FUNCTION_BLOCK FB84
TITLE =Move With Velocity
//*****************************************************************************
//* maxon motor ag
//* R&D
//* all rights reserved
//*****************************************************************************
//* Summary:  Move with target velocity
//*
//* Remarks:
//*
//* Created under: STEP7 REV5.2+SP1
//*****************************************************************************
//* History:
//* 19.05.2004 | INA   first release
//*
//*
//*****************************************************************************
//

AUTHOR:INA
FAMILY:ProVeloM
NAME:MoveWVel
VERSION:00.01


VAR_INPUT

Write : BOOL //A rising edge start the command

  NodeID : BYTE //Adress of the maxon device

  TargetVelocity : DINT //Target Velocity

END_VAR
VAR_OUTPUT
  Done : BOOL //Data valid flag is TRUE if data were available

  Err : BOOL //Error flag is TRUE if an Error has occured, see ErrNo for more details

  ErrNo : DINT //Contains detailed error information

END_VAR
VAR
  xEdgeMerker : BOOL //Edge Merker

  xEdgeFlag : BOOL //Edge Flag

  xStep : INT
  xMoveWithVelocity : WORD  := W#16#F
END_VAR

BEGIN

NETWORK
TITLE = Activate the service function
//

// SDO Write "Move With Velocity"

       U    #Write
       FP   #xEdgeFlag                   // recognize a positiv edge of the Read signal
       =    #xEdgeMerker                 // and set the xEdgeMerker for one cycle to true

       L    #xStep
       L    0
       ==I
       U    #xEdgeMerker
       SPB  nstp                         // iStep = 1 -> fnc1

       L    #xStep                       // jump list
       SPL  List
       SPA  rdef
       SPA  fnc1
       SPA  fncE
List  :SPA  rdef

rdef  :NOP  0
       R    #Done                        // reset Done
       R    #Err                         // reset Error
       L    0
       T    #xStep                       // iStep = 0
       SPA  end

fnc1  :NOP  0
       CALL FC13
         NodeID:=#NodeID
         Index:=DW#16#000060FF
         SubIndex:=DW#16#00000000
         ValueIn:=#TargetVelocity
         RET_VAL:=#Done
         Err:=#Err
         ErrNo:=#ErrNo

       L    1
       U    #Err
       SPB  fncE

       NOP  0
       CALL FC15
         NodeID:=#NodeID
         Index:=DW#16#00006040
         SubIndex:=DW#16#00000000
         ValueIn:=#xMoveWithVelocity
         RET_VAL:=#Done
         Err:=#Err
         ErrNo:=#ErrNo

fncE  :NOP  0
       L    0
       T    #xStep
       SPA  end

nstp  :NOP  0
       L    #xStep
       INC            1
       T    #xStep

end   :NOP  0
END_FUNCTION_BLOCK
